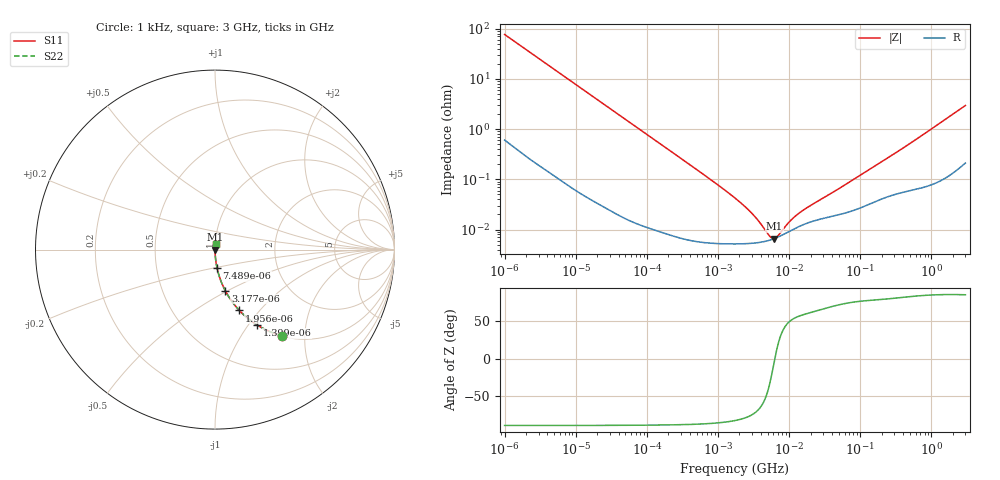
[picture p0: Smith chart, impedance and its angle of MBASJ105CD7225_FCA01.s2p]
! MBASJ105CD7225_FCA01  S-PARAMETER MODEL  ( Standard Model )
! Model Generated by TAIYO YUDEN Corporation (http://www.ty-top.com)
! Version 1.0
! TAIYO YUDEN Control No. 220901
! Copyright(c) 2022 TAIYO YUDEN CO.,LTD. All Rights Reserved.
! Product Description (link to TY-COMPAS)
! https://ds.yuden.co.jp/TYCOMPAS/or/detail?pn=MBASJ105CD7225KFCA01&u=M
! Products Name : Multilayer Ceramic Capacitors
! Characteristics :
!  Capacitance : 2.2 [uF] , Rated Voltage : 6.3 [V] , TCC : X7T
!  Case Size : 1.0 x 0.5 / 0.039 x 0.02 [mm/inch] , Thickness : 0.5 / 0.02 [mm/inch]
!  (Conditions: Temperature = 25 [degC] , DC Bias Voltage = 0 [V])
! External Node Assignments :
!  1  o---| |---o  2
! GND o---------o GND
! Frequency Range : 1kHz  -  3GHz  [ 401 STEP ]
# MHZ S RI R 50
! Freq[MHz].  S11 Real  S11 Imag  S21 Real  S21 Imag  S12 Real  S12 Imag  S22 Real  S22 Imag
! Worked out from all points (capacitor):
!   401 points, 1 kHz to 3 GHz, reference 50 ohm
!   read as one part in series: C = 2.07 uF near 1.077 kHz
!   lowest |Z| = 6.63 mohm at 6.153 MHz (marker M1)
!   series resonance near 6.288 MHz, so ESL is about 310 pH
!   S11 on the Smith chart (normalised r, x): 1 kHz: 1.01, -1.53; 1.399 kHz: 1.01, -1.10; 1.956 kHz: 1.01, -0.79; 3.177 kHz: 1.00, -0.49; 7.489 kHz: 1.00, -0.21; 3 GHz: 1.00, +0.06
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0.001  0.3713 -0.4792  0.6287 0.4792  0.6287 0.4792  0.3713 -0.4792
0.001399  0.2335 -0.4192  0.7665 0.4192  0.7665 0.4192  0.2335 -0.4192
0.001956  0.1358 -0.3389  0.8642 0.3389  0.8642 0.3389  0.1358 -0.3389
0.003177  0.0571 -0.2284  0.9429 0.2284  0.9429 0.2284  0.0571 -0.2284
0.004787  0.0265 -0.1569  0.9735 0.1569  0.9735 0.1569  0.0265 -0.1569
0.007489  0.0113 -0.1021  0.9887 0.1021  0.9887 0.1021  0.0113 -0.1021
0.01216  0.00455 -0.0635  0.9955 0.0635  0.9955 0.0635  0.00455 -0.0635
0.033275  0.00077 -0.0234  0.9992 0.0234  0.9992 0.0234  0.00077 -0.0234
0.147855  0.00012 -0.00531  0.9999 0.00531  0.9999 0.00531  0.00012 -0.00531
0.762639  5.49e-05 -0.00102  0.9999 0.00102  0.9999 0.00102  5.49e-05 -0.00102
1.732051  5.2e-05 -0.000422  0.9999 0.000422  0.9999 0.000422  5.2e-05 -0.000422
2.919173  5.33e-05 -0.000212  0.9999 0.000212  0.9999 0.000212  5.33e-05 -0.000212
4.566395  5.82e-05 -8.09e-05  0.9999 8.09e-05  0.9999 8.09e-05  5.82e-05 -8.09e-05
4.919932  5.97e-05 -6.14e-05  0.9999 6.14e-05  0.9999 6.14e-05  5.97e-05 -6.14e-05
6.153411  6.61e-05 -5.24e-06  0.9999 5.24e-06  0.9999 5.24e-06  6.61e-05 -5.24e-06
7.696136  7.59e-05 4.82e-05  0.9999 -4.82e-05  0.9999 -4.82e-05  7.59e-05 4.82e-05
8.291982  8e-05 6.55e-05  0.9999 -6.55e-05  0.9999 -6.55e-05  8e-05 6.55e-05
12.49624  0.000108 0.000157  0.9999 -0.000157  0.9999 -0.000157  0.000108 0.000157
21.06097  0.000145 0.000281  0.9999 -0.000281  0.9999 -0.000281  0.000145 0.000281
49.64928  0.000198 0.000618  0.9998 -0.000618  0.9998 -0.000618  0.000198 0.000618
256.0921  0.00047 0.00277  0.9995 -0.00277  0.9995 -0.00277  0.00047 0.00277
3000  0.00297 0.0293  0.997 -0.0293  0.997 -0.0293  0.00297 0.0293
